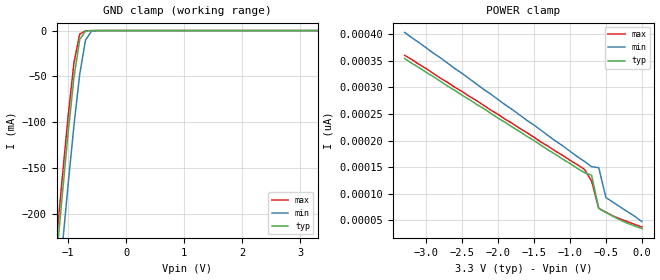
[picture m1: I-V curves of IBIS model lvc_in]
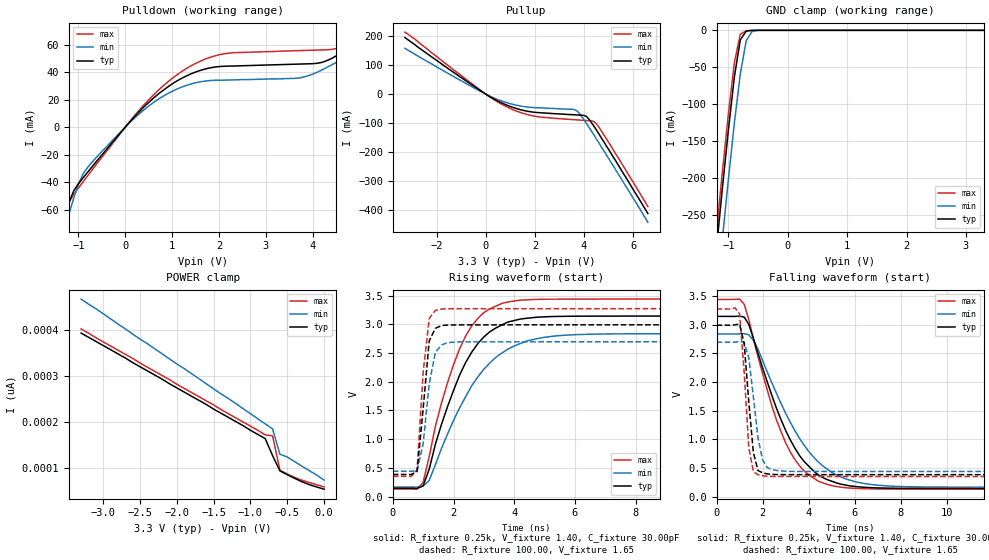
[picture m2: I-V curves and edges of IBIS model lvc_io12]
| IBIS file 162245xr.ibs created by s2ibis2 version 1.1
| North Carolina State University Electronics Research Laboratory  1995
[IBIS ver]   2.1
[File name]   162245xr.ibs
[File Rev]   1.0
[Date]   02/04/99 jbp
[Source]   Integrated Device Technology, Inc.
[Notes]   1.Temperatures: typ=25C, min=100C, max=0C 2.RRmp rates based
   on 50 ohm load.
[Disclaimer] Integrated Device Technology, Inc. ("IDT") hereby grants the
   user of this IBIS model a non-exclusive, nontransferable
   license to use this IBIS model under the following terms. The
   user is granted this license only to use the IBIS model and is
   not granted rights to sell, copy (except as needed to run the
   IBIS model), rent, lease or sub-license the IBIS model in
   whole or in part, or in modified form to anyone. The User may
   modify the IBIS model to suit its specific applications, but
   rights to derivative works and such modifications shall belong
   to IDT. This IBIS model is provided on an AS IS" basis and IDT
   makes absolutely no warranty with respect to the information
   contained herein. IDT DISCLAIMS AND CUSTOMER WAIVES ALL
   WARRANTIES, EXPRESS AND IMPLIED, INCLUDING WARRANTIES OF
   MERCHANTABILITY AND FITNESS FOR A PARTICULAR PURPOSE. THE
   ENTIRE RISK AS TO QUALITY AND PERFORMANCE IS WITH THE USER
   ACCORDINGLY, IN NO EVENT SHALL IDT BE LIABLE FOR ANY DIRECT OR
   INDIRECT DAMAGES, WHETHER IN CONTRACT OR TORT, INCLUDING ANY
   LOST PROFITS OR OTHER INCIDENTAL, CONSEQUENTIAL, EXEMPLARY, OR
   PUNITIVE DAMAGES ARISING OUT OF THE USE OR APPLICATION OF THE
   IBIS model. Further, IDT reserves the right to make changes
   without notice to any product herein to improve reliability,
   function, or design. IDT does not convey any license under
   patent rights or any other intellectual property rights,
   including those of third parties. IDT is not obligated to
   provide maintenance or support for the licensed IBIS model.
[Copyright]   Copyright 1997, Integrated Device Technology, Inc. all rights
   reserved
|   Component LVCR162245
[Component]   LVCR162245
[Manufacturer]   Integrated Device Technology
[Package]
| PA48
| variable   typ   min   max
R_pkg   6.50m   5.00m   10.00m
L_pkg   3.20nH   2.50nH   4.40nH
C_pkg   0.27pF   0.01pF   0.98pF
| PV48   typ   min   max
|R_pkg   6.5m   5.00m   10.00m
|L_pkg   4.75nH   3.82nH   6.72nH
|C_pkg   0.24pF   0.01pF   1.55pF
[Pin]  signal_name   model_name   R_pin   L_pin   C_pin
1   1DIR   lvc_in
2   1B1   lvc_io12
3   1B2   lvc_io12
4   GND   GND
5   1B3   lvc_io12
6   1B4   lvc_io12
7   VCC   POWER
8   1B5   lvc_io12
9   1B6   lvc_io12
10   GND   GND
11   1B7   lvc_io12
12   1B8   lvc_io12
13   2B1   lvc_io12
14   2B2   lvc_io12
15   GND   GND
16   2B3   lvc_io12
17   2B4   lvc_io12
18   VCC   POWER
19   2B5   lvc_io12
20   2B6   lvc_io12
21   GND   GND
22   2B7   lvc_io12
23   2B8   lvc_io12
24   2DIR   lvc_in
25   2OE_   lvc_in
26   2A8   lvc_io12
27   2A7   lvc_io12
28   GND   GND
29   2A6   lvc_io12
30   2A5   lvc_io12
31   VCC   POWER
32   2A4   lvc_io12
33   2A3   lvc_io12
34   GND   GND
35   2A2   lvc_io12
36   2A1   lvc_io12
37   1A8   lvc_io12
38   1A7   lvc_io12
39   GND   GND
40   1A6   lvc_io12
41   1A5   lvc_io12
42   VCC   POWER
43   1A4   lvc_io12
44   1A3   lvc_io12
45   GND   GND
46   1A2   lvc_io12
47   1A1   lvc_io12
48   1OE_   lvc_in
| Models and submodels in the file (2): lvc_in (Input), lvc_io12 (I/O)
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| in   in   dummy_model
| oe   oe
|   Model lvc_in
[Model]   lvc_in
Model_type   Input
Vinl =  0.800V
Vinh =  2.000V
C_comp   3.00pF   NA   NA
[Temperature Range]   25.00   100.00   0.000
[Voltage Range]   3.30V   3.00V   3.60V
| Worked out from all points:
|   GND clamp passes 1 mA (typ) near -0.70 V on its own axis
[GND_clamp]
| voltage   I(typ)   I(min)   I(max)
-3.3V     -1.806A    -1.858A    -1.789A
-1.2V     -248mA     -306mA     -229mA
-1.1V     -179mA     -236mA     -160mA
-1V       -112mA     -168mA     -93.56mA
-900mV    -51.39mA   -104mA     -35.36mA
-800mV    -9.697mA   -47.7mA    -3.786mA
-700mV    -714uA     -10.4mA    -348uA
-600mV    -52.42uA   -951uA     -8.225uA
-500mV    -126nA     -30.48uA   -10.89nA
3.3V      34.69pA    75.27pA    23pA
[POWER_clamp]
| voltage   I(typ)   I(min)   I(max)
-3.3V     354pA      403pA      360pA
-800mV    140pA      161pA      146pA
-700mV    135pA      151pA      124pA
-600mV    72.75pA    149pA      72.79pA
-500mV    65.09pA    93.05pA    65.39pA
-300mV    50.77pA    75.27pA    52.78pA
0V        34.68pA    47.91pA    37.83pA
|   Model lvc_io12
[Model]   lvc_io12
Model_type   I/O
Polarity   Non-Inverting
Enable   Active-High
Vinl =  0.000V
Vinh =  2.000V
Vmeas =  1.500V
C_comp   3.00pF   NA   NA
[Temperature Range]   25.00   100.00   0.000
[Voltage Range]   3.30V   3.00V   3.60V
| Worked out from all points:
|   slope of the pulldown table from 0 to 0.495 V, typ, clamps not added: 27.7 ohm
|   slope of the pullup table from 0 to 0.495 V, typ, clamps not added: 20.6 ohm
|   GND clamp passes 1 mA (typ) near -0.69 V on its own axis
|   rising waveform, R_fixture 0.25k, V_fixture 1.40, C_fixture 30.00pF: 20-80 % time 1.32ns typ, 1.65ns min, 1.15ns max; typ from 0.143 V to 3.15 V
|   rising waveform, R_fixture 100.00, V_fixture 1.65: 20-80 % time 273ps typ, 316ps min, 256ps max; typ from 0.384 V to 2.99 V
|   falling waveform, R_fixture 0.25k, V_fixture 1.40, C_fixture 30.00pF: 20-80 % time 1.8ns typ, 2.12ns min, 1.6ns max; typ from 3.15 V to 0.143 V
|   falling waveform, R_fixture 100.00, V_fixture 1.65: 20-80 % time 330ps typ, 417ps min, 289ps max; typ from 2.99 V to 0.384 V
[Pulldown]
| voltage   I(typ)   I(min)   I(max)
-3.3V     -330mA     -340mA     -326mA
-1.4V     -77.6mA    -87.8mA    -74.8mA
-1.3V     -65.6mA    -75.3mA    -63.5mA
-900mV    -36.9mA    -34mA      -39.8mA
47.68nV   1.93nA     1.67nA     2.11nA
900mV     29.1mA     24.3mA     32.7mA
1.7V      42.3mA     33.5mA     49.5mA
3.8V      46mA       36.4mA     55.8mA
4.5V      51.9mA     47.1mA     57.2mA
5.4V      72.8mA     65.6mA     76mA
5.8V      83.6mA     74.6mA     87.3mA
6.6V      106mA      93.6mA     112mA
[Pullup]
| voltage   I(typ)   I(min)   I(max)
-3.3V     195mA      158mA      214mA
-300mV    16.6mA     13.3mA     18.8mA
700mV     -32.2mA    -25.2mA    -37.1mA
1.3V      -50.8mA    -38.9mA    -59.8mA
1.9V      -61.5mA    -45.8mA    -74.3mA
3.5V      -70.5mA    -52mA      -87.3mA
3.7V      -71.4mA    -56.7mA    -88.4mA
4.1V      -76.8mA    -101mA     -90.7mA
4.4V      -110mA     -140mA     -94mA
4.5V      -123mA     -154mA     -102mA
5.1V      -204mA     -235mA     -179mA
6.6V      -411mA     -441mA     -387mA
[GND_clamp]
| voltage   I(typ)   I(min)   I(max)
-3.3V     -2.124A    -2.187A    -2.104A
-1.2V     -295mA     -364mA     -273mA
-1.1V     -213mA     -282mA     -191mA
-1V       -135mA     -202mA     -113mA
-900mV    -63.26mA   -126mA     -44.04mA
-800mV    -13.05mA   -59.39mA   -5.392mA
-700mV    -1.078mA   -14.09mA   -528uA
-600mV    -79.2uA    -1.428mA   -12.2uA
-500mV    -192nA     -46.42uA   -16.45nA
3.3V      54.14pA    104pA      44.85pA
[POWER_clamp]
| voltage   I(typ)   I(min)   I(max)
-3.3V     393pA      467pA      402pA
-800mV    164pA      196pA      172pA
-700mV    127pA      185pA      170pA
-600mV    93.79pA    130pA      95.18pA
-500mV    85.56pA    124pA      87.18pA
-300mV    70.17pA    104pA      73.5pA
0V        54.14pA    73.77pA    59.05pA
[Ramp]
| variable   typ   min   max
dV/dt_r   1.26/0.25n   1.02/0.31n   1.46/0.27n
dV/dt_f   1.06/0.42n   0.85/0.53n   1.24/0.40n
R_load = 50.00
[Rising Waveform]
R_fixture = 0.25k
V_fixture = 1.40
C_fixture = 30.00pF
R_dut = 7.00m
L_dut = 3.30nH
C_dut = 0.29pF
| time   V(typ)   V(min)   V(max)
0s        143mV      165mV      131mV
1ns       186mV      180mV      247mV
1.2ns     477mV      281mV      697mV
1.6ns     1.25V      835mV      1.621V
2.2ns     2.115V     1.543V     2.572V
2.8ns     2.664V     2.083V     3.102V
3.6ns     2.992V     2.502V     3.365V
4.4ns     3.105V     2.707V     3.426V
6ns       3.141V     2.819V     3.439V
19.8ns    3.145V     2.838V     3.44V
[Rising Waveform]
R_fixture = 100.00
V_fixture = 1.65
R_dut = 7.00m
L_dut = 3.30nH
C_dut = 0.29pF
| time   V(typ)   V(min)   V(max)
0s        384mV      440mV      352mV
600ps     383mV      439mV      349mV
800ps     433mV      450mV      461mV
1ns       1.525V     919mV      2.159V
1.2ns     2.71V      1.962V     3.103V
1.4ns     2.929V     2.506V     3.242V
1.6ns     2.978V     2.64V      3.265V
1.8ns     2.987V     2.68V      3.27V
2.2ns     2.99V      2.694V     3.271V
19.8ns    2.991V     2.695V     3.273V
[Falling Waveform]
R_fixture = 0.25k
V_fixture = 1.40
C_fixture = 30.00pF
R_dut = 7.00m
L_dut = 3.30nH
C_dut = 0.29pF
| time   V(typ)   V(min)   V(max)
0s        3.145V     2.838V     3.44V
1.2ns     3.133V     2.844V     3.356V
1.6ns     2.765V     2.728V     2.749V
2.4ns     1.769V     1.988V     1.587V
3ns       1.156V     1.455V     941mV
3.6ns     719mV      1.018V     540mV
4.4ns     384mV      611mV      274mV
5.6ns     203mV      311mV      157mV
7.4ns     149mV      188mV      133mV
19.8ns    143mV      165mV      131mV
[Falling Waveform]
R_fixture = 100.00
V_fixture = 1.65
R_dut = 7.00m
L_dut = 3.30nH
C_dut = 0.29pF
| time   V(typ)   V(min)   V(max)
0s        2.991V     2.695V     3.273V
1ns       3.011V     2.71V      3.192V
1.2ns     2.671V     2.688V     2.177V
1.4ns     1.652V     2.425V     856mV
1.6ns     769mV      1.742V     436mV
1.8ns     455mV      1.025V     384mV
2ns       417mV      641mV      366mV
2.2ns     398mV      509mV      356mV
2.8ns     385mV      450mV      353mV
19.8ns    384mV      440mV      352mV
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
